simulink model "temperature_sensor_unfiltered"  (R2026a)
settings: Solver=FixedStepAuto  StopTime=inf  EnableMultiTasking=on
libraries: arduinolib x1

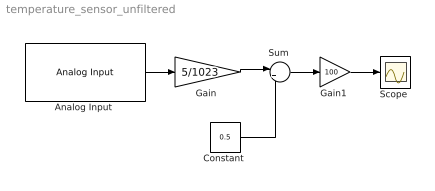
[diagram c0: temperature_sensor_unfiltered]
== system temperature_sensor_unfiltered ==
  "Analog Input " : arduinolib/Analog Input  pinNumber=4  ReadResultsOnly=off  ConversionTriggerSource=Software  ExternalTriggerType=uint32( 0 )  OutputDataType=uint16  EnableConversionCompleteNotify=off  EnableOuputStatus=off  SampleTime=0.01  blockPlatform=arduino
  "Constant " : Constant  Value=0.5
  "Gain " : Gain  Gain=5/1023
  "Gain1 " : Gain  Gain=100
  "Scope " : Scope
  "Sum " : Sum  Inputs=|+-
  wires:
  "Analog Input "/1 -> "Gain "/1
  "Gain "/1 -> "Sum "/1
  "Constant "/1 -> "Sum "/2
  "Sum "/1 -> "Gain1 "/1
  "Gain1 "/1 -> "Scope "/1
